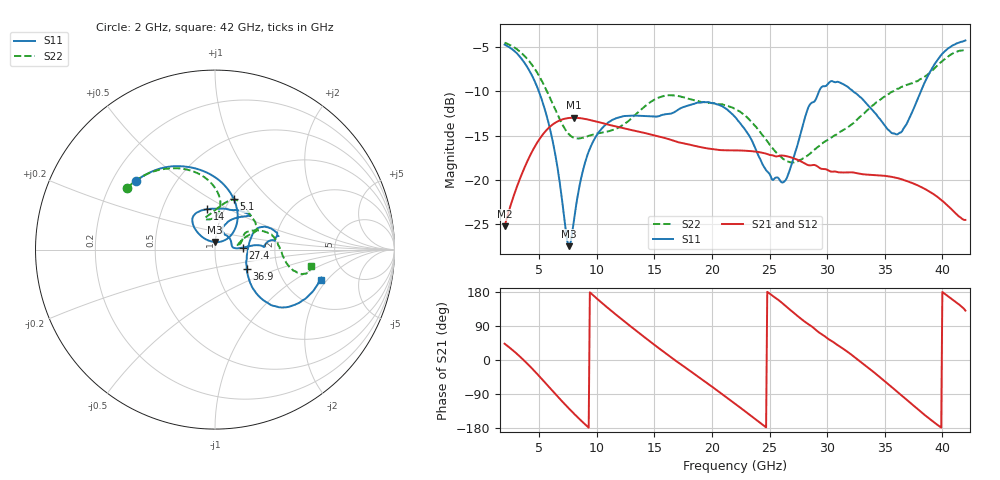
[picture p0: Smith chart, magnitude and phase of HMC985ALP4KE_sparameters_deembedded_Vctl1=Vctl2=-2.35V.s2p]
!s2p File: Measurements: S11, S21, S12, S22
# GHz S dB R 50.0
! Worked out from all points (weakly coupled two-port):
!   401 points, 2 GHz to 42 GHz, reference 50 ohm
!   highest |S21| = -12.98 dB at 8 GHz (marker M1); lowest = -25.3 dB at 2 GHz (marker M2)
!   lowest |S11| = -27.6 dB at 7.6 GHz (marker M3), VSWR 1.09, Z = 50 + j4.19 ohm
!   |S11| at or under -10 dB: 4.975 GHz to 29.29 GHz (24.32 GHz wide, 142 % of centre); 32.27 GHz to 38.12 GHz (5.858 GHz wide, 16.6 % of centre)
!   |S22| runs from -18.1 to -4.5 dB; largest |S21 - S12| = 0.00021
!   S11 on the Smith chart (normalised r, x): 2 GHz: 0.30, +0.35; 5.1 GHz: 1.03, +0.64; 14 GHz: 0.83, +0.40; 27.4 GHz: 1.36, +0.03; 36.9 GHz: 1.39, -0.31; 42 GHz: 3.21, -1.72
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2  -4.68 138.8  -25.29 43.0  -25.30 42.9  -4.46 145.1
3.5  -6.34 107.4  -19.36 4.2  -19.36 4.2  -5.68 119.5
5.1  -10.45 69.6  -15.27 -45.8  -15.27 -45.8  -8.49 94.0
6.3  -16.47 44.6  -13.63 -86.2  -13.64 -86.2  -11.77 83.2
7.6  -27.56 87.6  -13.01 -128.6  -13.02 -128.6  -14.88 90.3
8  -24.82 122.3  -12.98 -140.9  -12.99 -140.9  -15.26 95.3
8.7  -19.50 135.6  -13.06 -161.7  -13.06 -161.7  -15.29 103.1
10.7  -13.85 128.5  -13.66 144.0  -13.66 144.0  -14.61 106.9
14  -12.79 100.8  -14.67 63.5  -14.67 63.5  -11.89 80.6
15.4  -12.80 83.4  -15.13 30.9  -15.13 30.9  -10.68 71.5
19.1  -11.24 45.1  -16.34 -50.5  -16.35 -50.5  -11.21 44.1
22  -12.88 52.9  -16.69 -115.2  -16.70 -115.3  -11.98 24.4
25.3  -20.05 57.4  -17.26 168.5  -17.27 168.5  -16.53 17.8
26.4  -20.06 7.6  -17.32 142.3  -17.33 142.3  -17.85 11.1
27.4  -16.20 4.0  -17.74 116.9  -17.74 116.9  -17.96 8.3
28.7  -11.25 3.1  -18.36 87.7  -18.37 87.7  -16.81 12.8
31.1  -9.00 15.8  -19.19 35.5  -19.19 35.5  -14.61 28.0
33.3  -11.20 26.5  -19.43 -13.9  -19.43 -13.9  -12.38 26.2
35.4  -14.46 7.0  -19.66 -66.3  -19.66 -66.3  -10.24 17.8
36.9  -13.69 -31.7  -20.16 -105.0  -20.17 -105.0  -9.26 9.1
39.7  -6.19 -41.1  -22.09 -173.9  -22.10 -174.0  -6.92 -15.0
42  -4.21 -15.7  -24.58 130.3  -24.59 130.2  -5.33 -9.8
